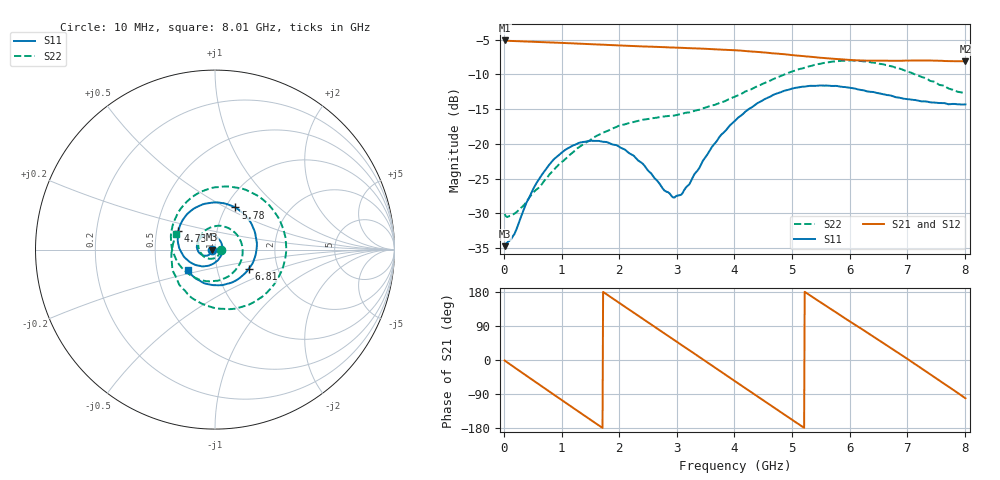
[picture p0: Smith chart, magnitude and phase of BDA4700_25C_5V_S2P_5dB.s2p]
!Agilent Technologies,E5071B,MY42404982,A.09.10
!Date: Mon Oct 20 13:28:24 2025
!Data & Calibration Information:
!Freq	S11:SOLT2(ON)	S21:SOLT2(ON)	S12:SOLT2(ON)	S22:SOLT2(ON)
# Hz S RI R 50
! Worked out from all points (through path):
!   801 points, 10 MHz to 8.01 GHz, reference 50 ohm
!   highest |S21| = -5.12 dB at 10 MHz (marker M1); lowest = -8.1 dB at 8.01 GHz (marker M2)
!   group delay of S21, straight-line fit = 284 ps
!   lowest |S11| = -34.7 dB at 10 MHz (marker M3), VSWR 1.04, Z = 48.2 - j0.109 ohm
!   |S11| at or under -10 dB: start of sweep to end of sweep
!   |S22| runs from -30.5 to -8.0 dB; largest |S21 - S12| = 0.0043
!   S11 on the Smith chart (normalised r, x): 10 MHz: 0.96, -0.00; 4.73 GHz: 0.65, +0.14; 5.78 GHz: 1.11, +0.56; 6.81 GHz: 1.42, -0.32; 8.01 GHz: 0.72, -0.17
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1e7  -0.0183 -0.00113  0.5544 -0.012  0.5543 -0.0126  0.0311 -0.0027
3.3e8  -0.0249 -0.0211  0.4457 -0.315  0.4456 -0.3155  0.021 -0.0288
7.2e8  -0.0553 -0.0344  0.128 -0.5226  0.1278 -0.5228  -0.0208 -0.0515
1.02e9  -0.0854 -0.0203  -0.1607 -0.507  -0.1608 -0.5075  -0.0667 -0.0341
1.35e9  -0.1014 0.0168  -0.4132 -0.3236  -0.4136 -0.3241  -0.0934 0.0285
1.64e9  -0.09 0.0543  -0.5136 -0.0719  -0.514 -0.072  -0.0681 0.0937
1.93e9  -0.0576 0.0795  -0.4746 0.192  -0.4748 0.1925  0.00293 0.131
2.32e9  -0.00326 0.0764  -0.2356 0.4455  -0.2354 0.4459  0.1121 0.0937
2.68e9  0.0341 0.0404  0.0787 0.4918  0.0786 0.4918  0.1544 -0.0156
2.97e9  0.041 -0.00532  0.3087 0.3834  0.3089 0.3829  0.1189 -0.1072
3.37e9  0.00949 -0.0644  0.4777 0.0846  0.4783 0.0845  -0.00163 -0.175
3.67e9  -0.0453 -0.0911  0.4474 -0.1705  0.4475 -0.1715  -0.11 -0.1569
4.01e9  -0.1237 -0.0787  0.2636 -0.3905  0.2639 -0.3903  -0.2067 -0.0723
4.36e9  -0.1905 -0.00975  -0.0169 -0.4595  -0.0172 -0.4605  -0.2459 0.0697
4.73e9  -0.2043 0.105  -0.2882 -0.3406  -0.2875 -0.3417  -0.1877 0.232
5.35e9  -0.0514 0.2563  -0.411 0.0959  -0.4113 0.095  0.1186 0.3451
5.78e9  0.1135 0.2349  -0.228 0.338  -0.2275 0.3381  0.3342 0.2065
6.2e9  0.2175 0.1106  0.0497 0.3944  0.0538 0.3949  0.3911 -0.051
6.68e9  0.2135 -0.067  0.3241 0.2276  0.3251 0.227  0.2222 -0.2892
6.81e9  0.1875 -0.1076  0.3667 0.1488  0.3679 0.1473  0.149 -0.3192
7.33e9  0.0369 -0.1983  0.3421 -0.2024  0.3419 -0.2034  -0.1398 -0.2604
8.01e9  -0.1532 -0.1163  -0.0746 -0.3848  -0.0744 -0.3851  -0.2164 0.0861
